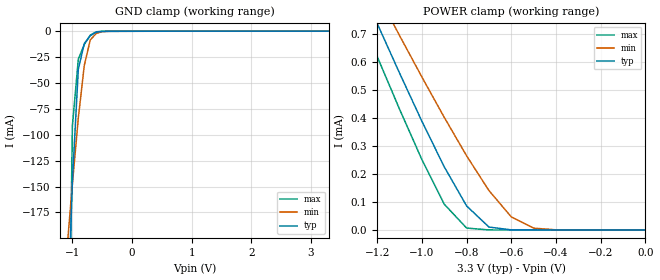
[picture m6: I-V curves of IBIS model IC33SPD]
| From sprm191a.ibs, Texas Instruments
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[Model]   IC33SPD
Model_type   Input
Polarity   Non-Inverting
| signals   A, Y
Vinl = 0.8V
Vinh = 2.0V
|   typ   min   max
C_comp   1.618p   1.587p   1.628p
|   typ   min   max
[Temperature Range]   25   -40   125
|   typ   min   max
[Voltage Range]   3.30V   3.00V   3.60V
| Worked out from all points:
|   GND clamp passes 1 mA (typ) near -0.60 V on its own axis
|   POWER clamp passes 1 mA (typ) near -1.35 V on its own axis
[GND_clamp]
|   Voltage   I(typ)   I(min)   I(max)
-3.3V     -5.028A    -1.945A    -16.49A
-1.1V     -316.5mA   -217.5mA   -508.5mA
-1V       -145.1mA   -147.6mA   -91.65mA
-900mV    -36.49mA   -83.63mA   -26.87mA
-800mV    -11.83mA   -32.98mA   -12.78mA
-700mV    -4.322mA   -8.36mA    -3.75mA
-600mV    -878.3uA   -2.067mA   -496uA
-500mV    -120.8uA   -393.4uA   -89.11uA
-400mV    -40.25uA   -66.09uA   -55.85uA
3.3V      100.4uA    51.97uA    176.9uA
[POWER_clamp]
|   Voltage   I(typ)   I(min)   I(max)
-3.3V     4.655mA    4.153mA    4.803mA
-1.3V     915.8uA    995.7uA    810uA
-1.2V     736.1uA    843.5uA    618.3uA
-1.1V     559.4uA    693uA      430.7uA
-1V       387.5uA    545.3uA    250.9uA
-900mV    225.1uA    401.4uA    91.98uA
-800mV    85.69uA    264.4uA    6.844uA
-700mV    10.39uA    140.5uA    74.52nA
-600mV    332.5nA    46.51uA    977pA
-500mV    8.571nA    6.514uA    355.3pA
-400mV    444.1pA    470.9nA    310.9pA
0V        1pA        1pA        1pA
